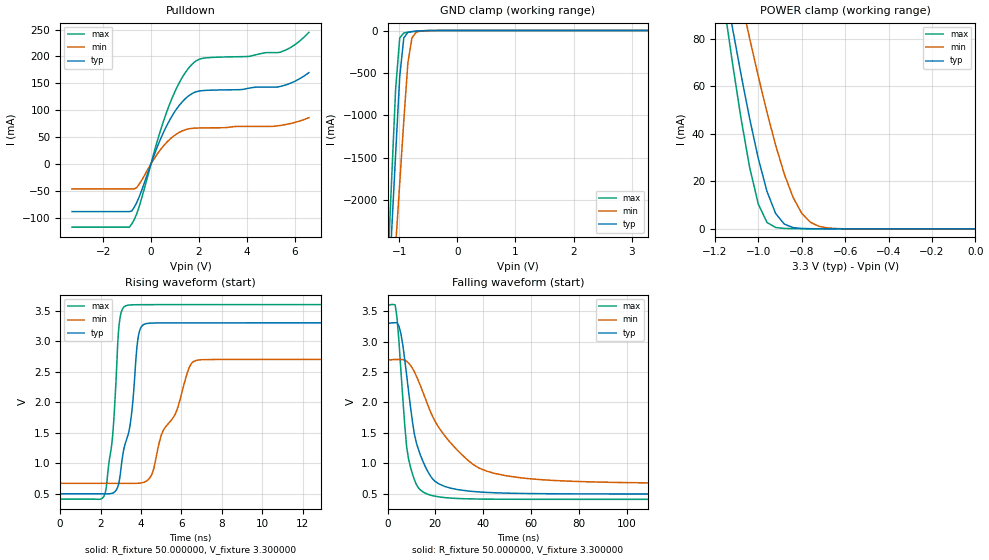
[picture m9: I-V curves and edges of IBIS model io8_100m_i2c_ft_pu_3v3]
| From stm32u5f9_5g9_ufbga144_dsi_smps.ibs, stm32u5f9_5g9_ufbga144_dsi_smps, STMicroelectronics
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|   Model io8_100m_i2c_ft_pu_3v3
[Model]  io8_100m_i2c_ft_pu_3v3
Model_type I/O_open_drain
Polarity   Non-Inverting
Enable   Active-Low
Vinl =   0.990000V
Vinh =   2.310000V
Vmeas =  1.650000V
Cref =   50.000000pF
Rref =   100.000000M
Vref =   1.650000V
C_comp   3.320400pF   3.288500pF   3.361100pF
[Temperature Range]   25.000000   0.140000k   -40.000000
[Pullup Reference]   3.300000V   2.700000V   3.600000V
[Pulldown Reference]   0.0V   0.0V   0.0V
[POWER Clamp Reference]   3.300000V   2.700000V   3.600000V
[GND Clamp Reference]   0.0V   0.0V   0.0V
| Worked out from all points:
|   slope of the pulldown table from 0 to 0.495 V, typ, clamps not added: 8.84 ohm
|   GND clamp passes 1 mA (typ) near -0.51 V on its own axis
|   POWER clamp passes 1 mA (typ) near -0.85 V on its own axis
|   rising waveform, R_fixture 50.000000, V_fixture 3.300000: 20-80 % time 691ps typ, 1.39ns min, 417ps max; typ from 0.496 V to 3.3 V
|   falling waveform, R_fixture 50.000000, V_fixture 3.300000: 20-80 % time 7.47ns typ, 19.4ns min, 4.08ns max; typ from 3.3 V to 0.496 V
[Pulldown]
|Voltage   I(typ)   I(min)   I(max)
-3.3V     -88.62mA   -46.48mA   -117.6mA
-900mV    -88.62mA   -46.48mA   -117.6mA
-700mV    -80.76mA   -46.48mA   -103.5mA
-500mV    -62.15mA   -38.24mA   -80.45mA
300mV     35.76mA    20.75mA    48.1mA
800mV     83.04mA    46.39mA    113.4mA
1.3V      115.2mA    61.33mA    160.4mA
1.8V      132.8mA    66.57mA    188.9mA
2.3V      136.9mA    67.16mA    197.4mA
5.4V      144.2mA    71.57mA    207.9mA
6V        153.5mA    77.1mA     221.4mA
6.6V      169.9mA    86.1mA     244.9mA
[GND_clamp]
|Voltage   I(typ)   I(min)   I(max)
-3.3V     -9.848A    -9.957A    -9.458A
-1.2V     -3.312A    -4.013A    -2.863A
-1.13V    -2.381A    -3.274A    -1.769A
-1.06V    -1.452A    -2.535A    -684.7mA
-990mV    -542.9mA   -1.798A    -88.02mA
-920mV    -87.11mA   -1.064A    -28.44mA
-850mV    -22.1mA    -382.4mA   -19.61mA
-780mV    -11.97mA   -86.98mA   -13.71mA
-710mV    -7.619mA   -22.26mA   -8.745mA
-640mV    -4.493mA   -7.773mA   -4.817mA
-360mV    -31.22uA   -172.6uA   -8.607uA
3.28V     0A         15.66nA    -5.841nA
[POWER_clamp]
|Voltage   I(typ)   I(min)   I(max)
-3.28V    1.355A     1.167A     1.665A
-1.16V    105.8mA    131.6mA    95.87mA
-1.12V    85.08mA    114mA      70.45mA
-1.08V    65.19mA    96.88mA    46.75mA
-1.04V    46.48mA    80.2mA     25.96mA
-1V       29.64mA    64.18mA    10.49mA
-960mV    15.81mA    49.06mA    2.743mA
-920mV    6.481mA    35.16mA    612.9uA
-840mV    578.2uA    13.29mA    138.5uA
-760mV    94.37uA    2.807mA    98.57uA
-640mV    40.55uA    159.2uA    59.97uA
0V        0A         19.29nA    0A
[Ramp]
| variable   typ   min   max
dV/dt_r  1.68220/0.76907n   1.21922/1.44451n   1.91462/0.52606n
dV/dt_f  1.68220/7.44931n   1.21922/19.37083n   1.91462/4.07072n
R_load = 50.000000
[Rising Waveform]
R_fixture= 50.000000
V_fixture= 3.300000
V_fixture_min= 2.700000
V_fixture_max= 3.600000
|time   V(typ)   V(min)   V(max)
0s        496.3mV    668mV      409mV
2.202ns   496.1mV    667.9mV    483.8mV
2.603ns   507.8mV    667.6mV    1.471V
2.923ns   699.8mV    667.3mV    3.284V
3.243ns   1.342V     667.1mV    3.578V
3.524ns   1.78V      667.2mV    3.594V
3.844ns   3.027V     668.1mV    3.596V
4.164ns   3.277V     688.2mV    3.597V
6.727ns   3.299V     2.682V     3.598V
19.94ns   3.3V       2.7V       3.6V
[Falling Waveform]
R_fixture= 50.000000
V_fixture= 3.300000
V_fixture_min= 2.700000
V_fixture_max= 3.600000
|time   V(typ)   V(min)   V(max)
0s        3.3V       2.7V       3.6V
3.203ns   3.309V     2.706V     3.603V
5.606ns   3.127V     2.706V     2.517V
8.008ns   2.444V     2.676V     1.266V
9.61ns    1.929V     2.61V      937.3mV
12.81ns   1.24V      2.365V     604.1mV
19.22ns   729.4mV    1.741V     465.6mV
37.64ns   532.1mV    936.9mV    414.1mV
64.06ns   501.8mV    732.4mV    409.3mV
398.8ns   496.3mV    668mV      409mV
